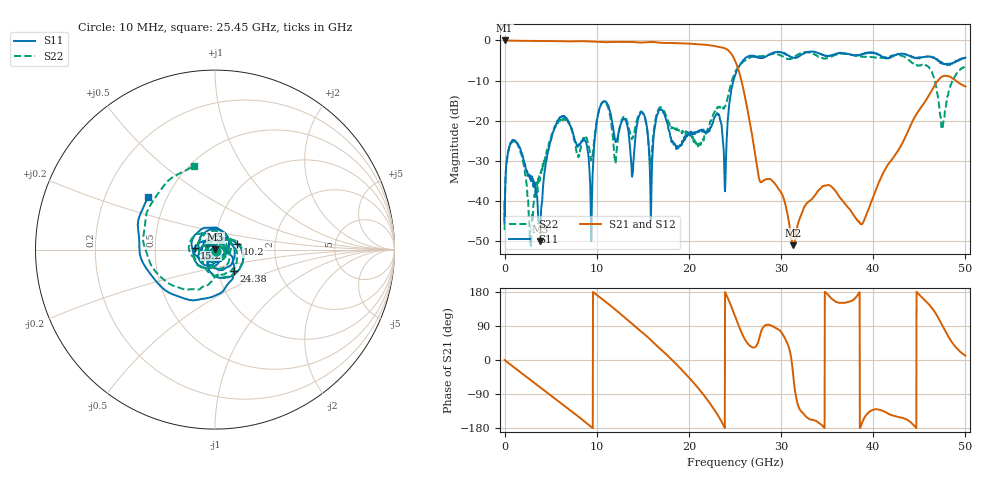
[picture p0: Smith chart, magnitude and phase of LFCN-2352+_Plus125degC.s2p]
! Mini-Circuits
! S2P DATA File Format
! Type: LOW PASS FILTER
! Model: LFCN-2352+
! All S Parameters are in dB deg format
! TEST CONDITIONS: INPUT POWER = 0 dBm - +125 deg C
# MHZ S DB R 50
!Frequency  S11 dB  S11 DEG  S21 dB  S21 DEG  S12 dB  S12 DEG  S22 dB  S22 DEG
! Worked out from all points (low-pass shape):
!   2006 points, 10 MHz to 50 GHz, reference 50 ohm
!   highest |S21| = -0.02 dB at 10 MHz (marker M1); lowest = -51.0 dB at 31.35 GHz (marker M2)
!   |S21| within 3 dB of the highest: start of sweep to 24.5 GHz
!   lowest |S11| = -50.0 dB at 3.875 GHz (marker M3), VSWR 1.01, Z = 50.2 + j0.216 ohm
!   |S11| at or under -10 dB: start of sweep to 24.83 GHz
!   |S22| runs from -51.2 to -2.9 dB; largest |S21 - S12| = 0.0028
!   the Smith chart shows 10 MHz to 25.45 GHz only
!   S11 on the Smith chart (normalised r, x): 10 MHz: 1.01, -0.01; 10.2 GHz: 1.28, +0.08; 15.2 GHz: 0.80, +0.02; 24.38 GHz: 1.20, -0.29; 25.45 GHz: 0.39, +0.30
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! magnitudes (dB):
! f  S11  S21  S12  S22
! 10 MHz  -40.0  0.0  0.0  -40.4
! 1.1 GHz  -24.9  -0.1  -0.1  -25.1
! 2.85 GHz  -34.2  -0.1  -0.2  -50.8
! 3.875 GHz  -50.0  -0.2  -0.2  -33.9
! 5.725 GHz  -20.0  -0.2  -0.2  -20.6
! 8.35 GHz  -25.0  -0.2  -0.2  -26.0
! 9.4 GHz  -49.9  -0.3  -0.3  -29.9
! 10.2 GHz  -17.9  -0.4  -0.4  -17.8
! 13.85 GHz  -33.9  -0.4  -0.4  -24.3
! 15.2 GHz  -18.9  -0.5  -0.5  -19.1
! 15.88 GHz  -44.9  -0.4  -0.4  -31.1
! 16.68 GHz  -17.9  -0.5  -0.5  -17.4
! 23.88 GHz  -35.7  -2.0  -2.0  -16.5
! 24.38 GHz  -16.1  -2.7  -2.7  -12.5
! 25.02 GHz  -8.7  -5.1  -5.1  -7.8
! 25.45 GHz  -6.5  -7.9  -7.9  -6.4
! 31.35 GHz  -4.3  -51.0  -50.9  -4.3
! 33.35 GHz  -2.8  -39.5  -39.5  -3.2
! 38.77 GHz  -3.5  -45.7  -45.7  -4.0
! 41.67 GHz  -4.4  -30.7  -30.7  -4.0
! 47.5 GHz  -5.7  -9.0  -9.0  -21.6
! 50 GHz  -4.3  -11.5  -11.5  -6.6
